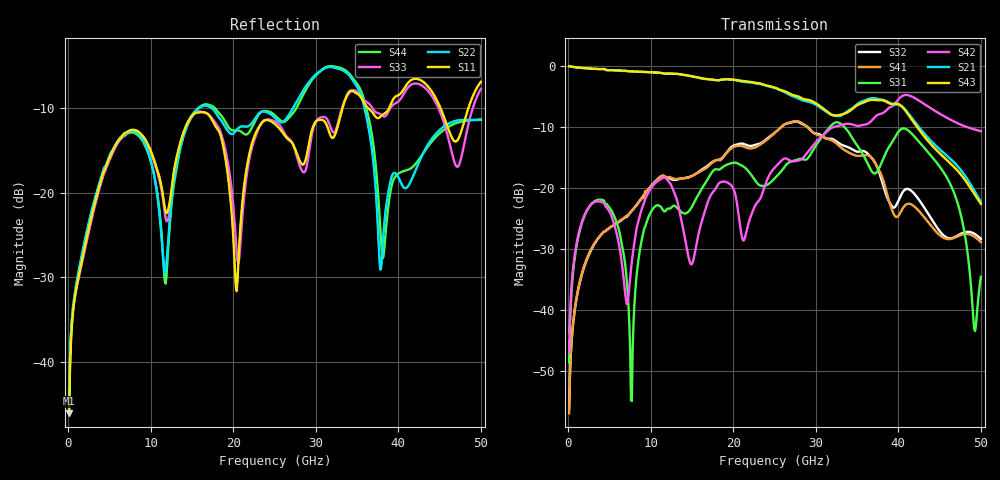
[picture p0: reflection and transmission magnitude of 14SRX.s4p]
! DAC39RF10ACK
! 256-pin FCBGA package
! Texas Instruments 8/20/2022
! Single-ended  S-parameters
! PORT#  PORT_NAME  NET_NAME
! PORT1:  xSRXN.DIEBUMP  xSRXN
! PORT2:  xSRXN.BGA  xSRXN
! PORT3:  xSRXP.DIEBUMP  xSRXP
! PORT4:  xSRXP.BGA  xSRXP
! Touchstone Ver. 1.0
! Number of ports is 4
# Hz	S	MA	R	50.000000
! SCATTERING PARAMETERS  :
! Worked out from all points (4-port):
!   500 points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, 100 MHz to 50 GHz, reference 50 ohm
!   strongest paths, dB at 100 MHz, 12.6 GHz, 25.1 GHz, 37.6 GHz, 50 GHz:
!     S43: 0.0, -1.2, -3.6, -5.6, -22.6
!     S21: 0.0, -1.2, -3.6, -5.4, -22.3
!     S42: -47.0, -19.9, -16.5, -7.9, -10.7
!     S31: -48.5, -23.0, -18.3, -16.9, -34.5
!     S41: -56.9, -18.4, -10.9, -16.9, -28.8
!     S32: -56.0, -18.6, -10.9, -17.1, -28.3
!   lowest |S11| = -46.1 dB at 100 MHz (marker M1), VSWR 1.01, Z = 50.4 + j0.311 ohm
!   |S11| at or under -10 dB: start of sweep to 33.24 GHz; 36.34 GHz to 38.89 GHz (2.544 GHz wide, 6.76 % of centre); 45.1 GHz to 48.49 GHz (3.386 GHz wide, 7.24 % of centre)
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1e8  0.004967 38.4  0.9953 -2.7  0.003891 83.9  0.00159 -100.8
     0.9958 -2.7  0.00568 40.9  0.001515 -100.0  0.004531 82.5
     0.003776 84.3  0.001585 -100.9  0.005351 41.0  0.9944 -2.8
     0.001437 -99.6  0.004487 82.9  0.9957 -2.6  0.005654 40.4
3.7e9  0.1063 13.1  0.9436 -89.4  0.08051 -5.4  0.03956 168.4
       0.9432 -89.2  0.1112 -27.9  0.03935 168.6  0.07815 3.2
       0.08052 -5.3  0.0394 168.8  0.1021 13.7  0.9429 -88.6
       0.03973 168.1  0.07799 3.3  0.9425 -88.5  0.1073 -27.6
7.4e9  0.2329 -65.9  0.902 -176.7  0.007589 -90.4  0.0618 89.8
       0.9033 -176.5  0.2305 -108.2  0.06176 92.1  0.01535 157.5
       0.007643 -91.4  0.06168 92.0  0.2293 -65.2  0.901 -175.4
       0.06212 90.4  0.01569 155.7  0.9046 -175.2  0.226 -106.9
1.48e10  0.2766 -92.9  0.8255 6.5  0.066 168.2  0.1248 -90.5
         0.8254 6.6  0.277 -77.5  0.124 -87.2  0.02113 18.1
         0.06724 167.9  0.1245 -87.0  0.2734 -89.2  0.8251 9.3
         0.1236 -90.0  0.02411 18.4  0.8276 9.3  0.2716 -76.5
2.26e10  0.2185 -67.5  0.7261 -178.5  0.1153 -158.4  0.2164 81.0
         0.7219 -179.0  0.2716 -122.7  0.2241 83.0  0.07134 49.7
         0.1167 -158.1  0.2255 83.3  0.2089 -59.0  0.7354 -174.4
         0.2148 80.8  0.07102 49.8  0.73 -174.7  0.2621 -120.3
2.96e10  0.2405 -85.7  0.4947 14.0  0.2012 -165.0  0.2848 -126.8
         0.4963 14.0  0.4774 -138.3  0.292 -120.4  0.2209 177.6
         0.202 -165.3  0.288 -120.5  0.2301 -77.5  0.5095 17.9
         0.2871 -126.8  0.2206 177.5  0.5126 17.8  0.4685 -135.4
5e10  0.4518 -99.1  0.0799 -70.9  0.03375 -160.0  0.03629 168.7
      0.07714 -87.0  0.269 -142.4  0.04017 -166.5  0.2861 -27.1
      0.01885 -155.4  0.03846 178.7  0.4101 -87.5  0.08103 -63.0
      0.0362 -167.5  0.2924 -27.0  0.07428 -56.2  0.2707 -142.5
